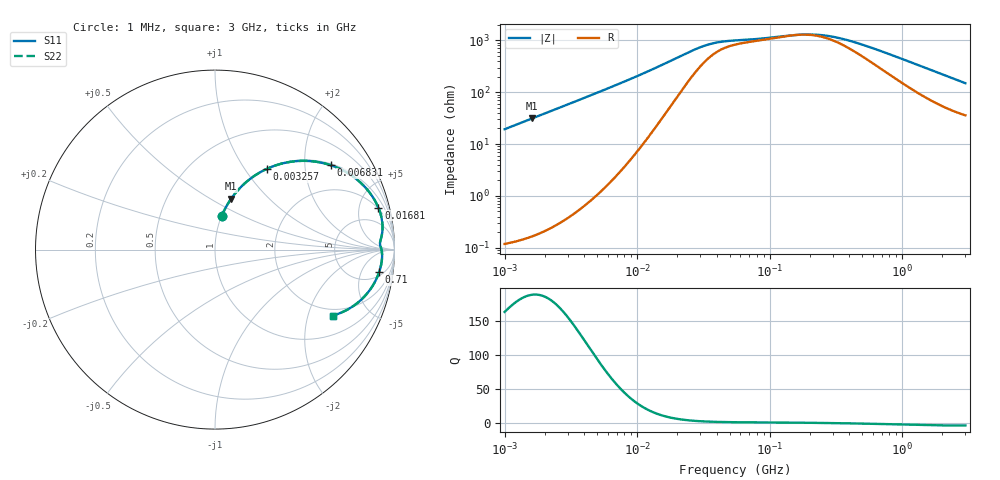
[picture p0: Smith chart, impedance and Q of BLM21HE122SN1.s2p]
! BLM21HE122SN1
# Hz S RI R 50
!Freq.(Hz) S11(Real) S11(Imag) S21(Real) S21(Imag) S12(Real) S12(Imag) S22(Real) S22(Imag)
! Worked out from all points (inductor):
!   401 points, 1 MHz to 3 GHz, reference 50 ohm
!   read as one part in series: L = 3.08 uH near 1.041 MHz
!   highest Q = 189 at 1.617 MHz (marker M1), where L = 3.08 uH
!   self-resonance near 161.3 MHz
!   S11 on the Smith chart (normalised r, x): 1 MHz: 1.00, +0.39; 3.257 MHz: 1.01, +1.27; 6.831 MHz: 1.05, +2.72; 16.81 MHz: 1.86, +7.45; 710 MHz: 6, -11; 3 GHz: 1.72, -2.91
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1000000  0.0371 0.1859  0.9629 -0.1859  0.9629 -0.1859  0.0371 0.1859
1616692  0.0904 0.2841  0.9096 -0.2841  0.9096 -0.2841  0.0904 0.2841
2317916  0.1693 0.3723  0.8307 -0.3723  0.8307 -0.3723  0.1693 0.3723
3257432  0.2877 0.4493  0.7123 -0.4493  0.7123 -0.4493  0.2877 0.4493
3823119  0.3582 0.4756  0.6418 -0.4756  0.6418 -0.4756  0.3582 0.4756
5161903  0.5067 0.4944  0.4933 -0.4944  0.4933 -0.4944  0.5067 0.4944
6831390  0.6459 0.4698  0.3541 -0.4698  0.3541 -0.4698  0.6459 0.4698
9992459  0.799 0.3836  0.201 -0.3836  0.201 -0.3836  0.799 0.3836
1.461624e7  0.8909 0.2733  0.1091 -0.2733  0.1091 -0.2733  0.8909 0.2733
1.681455e7  0.9102 0.234  0.0898 -0.234  0.0898 -0.234  0.9102 0.234
2.664524e7  0.9335 0.1278  0.0665 -0.1278  0.0665 -0.1278  0.9335 0.1278
3.320783e7  0.9315 0.0929  0.0685 -0.0929  0.0685 -0.0929  0.9315 0.0929
4.138676e7  0.9266 0.068  0.0734 -0.068  0.0734 -0.068  0.9266 0.068
5.477226e7  0.921 0.0474  0.079 -0.0474  0.079 -0.0474  0.921 0.0474
1.550909e8  0.9271 0.00203  0.0729 -0.00203  0.0729 -0.00203  0.9271 0.00203
2.094008e8  0.9301 -0.0146  0.0699 0.0146  0.0699 0.0146  0.9301 -0.0146
2.662515e8  0.9311 -0.0302  0.0689 0.0302  0.0689 0.0302  0.9311 -0.0302
3.453811e8  0.9305 -0.0496  0.0695 0.0496  0.0695 0.0496  0.9305 -0.0496
7.099691e8  0.9145 -0.1254  0.0855 0.1254  0.0855 0.1254  0.9145 -0.1254
8.005644e8  0.9084 -0.1422  0.0916 0.1422  0.0916 0.1422  0.9084 -0.1422
1.613037e9  0.8287 -0.2654  0.1713 0.2654  0.1713 0.2654  0.8287 -0.2654
3e9  0.6568 -0.3672  0.3432 0.3672  0.3432 0.3672  0.6568 -0.3672
